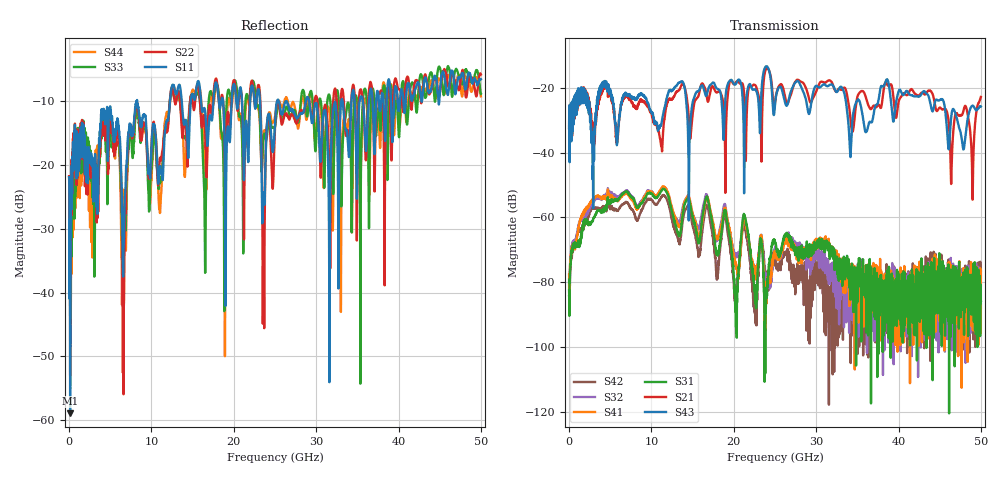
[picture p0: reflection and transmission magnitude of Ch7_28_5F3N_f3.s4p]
!Agilent Technologies,N5247A,US51170199,A.09.90.13
!Agilent N5247A: A.09.90.13
!Date: Wednesday, December 09, 2015 09:22:14
!Correction: S11(Full 4 Port(1,2,3,4))
!S12(Full 4 Port(1,2,3,4))
!S13(Full 4 Port(1,2,3,4))
!S14(Full 4 Port(1,2,3,4))
!S21(Full 4 Port(1,2,3,4))
!S22(Full 4 Port(1,2,3,4))
!S23(Full 4 Port(1,2,3,4))
!S24(Full 4 Port(1,2,3,4))
!S31(Full 4 Port(1,2,3,4))
!S32(Full 4 Port(1,2,3,4))
!S33(Full 4 Port(1,2,3,4))
!S34(Full 4 Port(1,2,3,4))
!S41(Full 4 Port(1,2,3,4))
!S42(Full 4 Port(1,2,3,4))
!S43(Full 4 Port(1,2,3,4))
!S44(Full 4 Port(1,2,3,4))
!S4P File: Measurements: <S11,S12,S13,S14>,
!<S21,S22,S23,S24>,
!<S31,S32,S33,S34>,
!<S41,S42,S43,S44>:
# Hz S  dB  R 50
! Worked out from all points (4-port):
!   3201 points, 10 MHz to 50 GHz, reference 50 ohm
!   strongest paths, dB at 10 MHz, 12.51 GHz, 25 GHz, 37.5 GHz, 50 GHz:
!     S43: -32.5, -20.9, -25.3, -24.7, -25.8
!     S21: -32.5, -23.5, -24.6, -25.4, -22.9
!     S31: -82.5, -58.3, -68.0, -90.5, -85.7
!     S41: -77.7, -57.0, -70.6, -83.6, -77.2
!     S32: -84.3, -57.4, -69.4, -90.2, -88.1
!     S42: -79.1, -60.7, -73.5, -87.3, -76.5
!   lowest |S11| = -58.9 dB at 135 MHz (marker M1), VSWR 1.00, Z = 50 + j0.104 ohm
!   |S11| at or under -10 dB: start of sweep to 8.239 GHz; 8.268 GHz to 12.26 GHz (3.992 GHz wide, 38.9 % of centre); 29.15 GHz to 33.06 GHz (3.909 GHz wide, 12.6 % of centre)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
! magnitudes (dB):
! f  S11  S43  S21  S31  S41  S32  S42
! 10 MHz  -21.9  -32.5  -32.5  -82.5  -77.7  -84.3  -79.1
! 135 MHz  -58.9  -33.0  -32.8  -76.2  -74.4  -74.0  -76.5
! 11.48 GHz  -19.1  -27.4  -31.5  -51.2  -50.4  -51.0  -53.2
! 20.29 GHz  -9.8  -18.7  -18.3  -87.0  -74.4  -71.5  -82.4
! 21.27 GHz  -20.9  -45.3  -22.6  -59.3  -60.3  -59.6  -62.0
! 23.63 GHz  -24.5  -15.1  -18.0  -78.5  -77.7  -73.6  -71.8
! 50 GHz  -6.6  -25.8  -22.9  -85.7  -77.2  -88.1  -76.5
